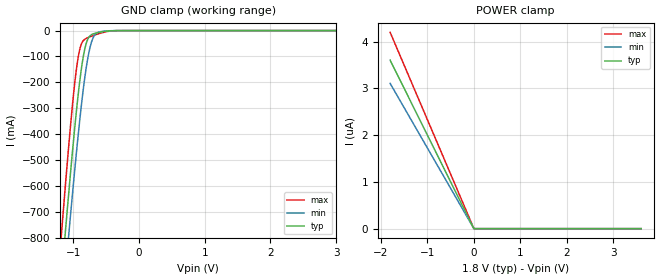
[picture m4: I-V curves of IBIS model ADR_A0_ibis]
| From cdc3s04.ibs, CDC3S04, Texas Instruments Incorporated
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|   1.8V  INPUT model
[Model]   ADR_A0_ibis
Model_type   Input
Vinl = 630.000mV
Vinh = 1.170V
|   typ   min   max
C_comp   798.1fF   773.9fF   816.4fF
[Voltage Range]   1.800V   1.650V   1.950V
[Temperature Range]   32.0   85.0   -40.0
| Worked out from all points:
|   GND clamp passes 1 mA (typ) near -0.43 V on its own axis
[GND Clamp]
|   Voltage   I(typ)   I(min)   I(max)
-1.8V     -2.926A    -3.001A    -2.86A
-1.192V   -994.5mA   -1.145A    -824.8mA
-1.173V   -934.9mA   -1.088A    -762.6mA
-1.129V   -803mA     -960.3mA   -625.3mA
-1.088V   -681.5mA   -842.1mA   -500.1mA
-1.055V   -588mA     -750.6mA   -405.3mA
-974.5mV  -366.7mA   -529.5mA   -195mA
-917.8mV  -230mA     -384.8mA   -92.21mA
-821.9mV  -67.73mA   -176mA     -33.07mA
-719.3mV  -15.33mA   -41.56mA   -21.34mA
-451.4mV  -1.28mA    -680.6uA   -2.377mA
3.599V    3.602uA    2.85uA     4.546uA
[POWER Clamp]
|   Voltage   I(typ)   I(min)   I(max)
-1.8V     3.602uA    3.106uA    4.195uA
-1.793V   3.584uA    3.09uA     4.176uA
0V        17.34pA    97.71pA    -32.05pA
3.599V    0A         0A         -40pA
